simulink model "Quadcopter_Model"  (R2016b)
settings: Solver=VariableStepAuto  StartTime=0.0  StopTime=10.0  RelTol=1e-3
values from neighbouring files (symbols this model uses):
  g = 9.81    [modelParameters.m]
  If = 0.511    [modelParameters.m]
  Jreq = 4.2012e-05    [modelParameters.m]
  Jxx = 0.0218    [modelParameters.m]
  Jyy = 0.0277    [modelParameters.m]
  Jzz = 0.0332    [modelParameters.m]
  Kd = 1.8087e-07    [modelParameters.m]
  Kq = 96.3422    [modelParameters.m]
  Kt = 8.1558*10^-6    (= 8.1558e-06)    [modelParameters.m]
  Kv = 96.3422    [modelParameters.m]
  m = 1.19    [modelParameters.m]
  Pmax = 0.80    (= 0.8)    [modelParameters.m]
  Pmin = 0.40    (= 0.4)    [modelParameters.m]
  rhx = 0.016    [modelParameters.m]
  rhy = 0.016    [modelParameters.m]
  rhz = 0.003    [modelParameters.m]
  Rm = 0.2308    [modelParameters.m]
  Vb = 11.1    [modelParameters.m]

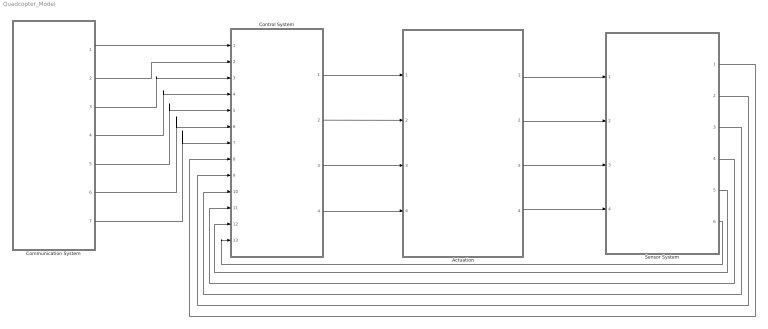
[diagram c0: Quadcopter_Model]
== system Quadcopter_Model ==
  Actuation : Subsystem
  Communication System : Subsystem
  Control System : Subsystem
  Sensor System : Subsystem
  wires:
  Control System/1(Rotor 0 Duty Cycle) -> Actuation/1(Rotor 0 Duty Cycle)
  Sensor System/6(Yaw rate (psi dot)) -> Control System/13(Yaw rate (psi dot))
  Sensor System/5(Roll rate (theta dot)) -> Control System/12(Roll rate (theta dot))
  Sensor System/4(Pitch rate (phi dot)) -> Control System/11(Pitch rate (phi dot))
  Sensor System/3(Yaw (psi)) -> Control System/10(Yaw (psi))
  Sensor System/2(Roll (theta)) -> Control System/9(Roll (theta))
  Sensor System/1(Pitch (phi)) -> Control System/8(Pitch (phi))
  Communication System/1(x_position) -> Control System/1(x position)
  Communication System/2(y_position) -> Control System/2(y position)
  Communication System/3(z_position) -> Control System/3(z position)
  Communication System/4(x_setpoint) -> Control System/4(x setpoint)
  Communication System/5(y_setpoint) -> Control System/5(y setpoint)
  Communication System/6(z_setpoint) -> Control System/6(z setpoint)
  Communication System/7(yaw_setpoint) -> Control System/7("Yaw setpoint ")
  Control System/2(Rotor 1 Duty Cycle) -> Actuation/2(Rotor 1 Duty Cycle)
  Control System/3(Rotor 2 Duty Cycle) -> Actuation/3(Rotor 2 Duty Cycle)
  Control System/4(Rotor 3 Duty Cycle) -> Actuation/4(Rotor 3 Duty Cycle)
  Actuation/1(B_omega) -> Sensor System/1(B_omega)
  Actuation/2(euler_angles) -> Sensor System/2(euler_angles)
  Actuation/3(B_vo) -> Sensor System/3(B_vo)
  Actuation/4(E_ro) -> Sensor System/4(E_ro)

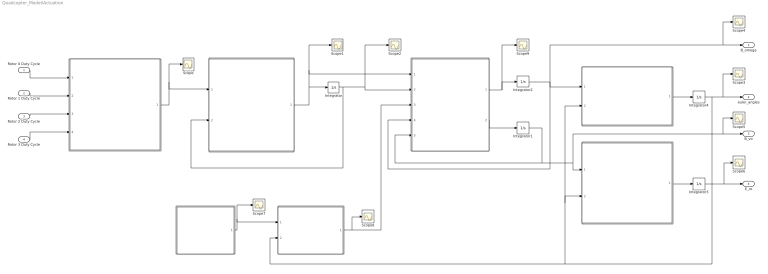
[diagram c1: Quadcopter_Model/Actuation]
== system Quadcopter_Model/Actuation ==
  Rotor 0 Duty Cycle : Inport
  Rotor 1 Duty Cycle : Inport  Port=2
  Rotor 2 Duty Cycle : Inport  Port=3
  Rotor 3 Duty Cycle : Inport  Port=4
  " " : MATLAB Function  TreatAsAtomicUnit=on
  " " : MATLAB Function  TreatAsAtomicUnit=on
  " " : MATLAB Function  TreatAsAtomicUnit=on
  " " : MATLAB Function  TreatAsAtomicUnit=on
  " " : MATLAB Function  TreatAsAtomicUnit=on
  " " : MATLAB Function  TreatAsAtomicUnit=on
  " " : MATLAB Function  TreatAsAtomicUnit=on
  Integrator{,1..3} (4 alike) : Integrator
  Integrator4 : Integrator  ContinuousStateAttributes=['phi' 'theta' 'psi']
  Scope{,1..9} (10 alike) : Scope
  B_omega : Outport
  euler_angles : Outport  Port=2
  B_vo : Outport  Port=3
  E_ro : Outport  Port=4
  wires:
  Rotor 3 Duty Cycle/1 -> " "/4(rotor_3_duty_cycle)
  Rotor 2 Duty Cycle/1 -> " "/3(rotor_2_duty_cycle)
  Rotor 1 Duty Cycle/1 -> " "/2(rotor_1_duty_cycle)
  Rotor 0 Duty Cycle/1 -> " "/1(rotor_0_duty_cycle)
  " "/1(Vb_eff) -> Scope/1, " "/1(Vb_eff)
  " "/1(angular_acceleration) -> Integrator/1, Scope1/1, " "/1(angular_acceleration)
  Integrator/1 -> Scope2/1, " "/2(angular_velocity), " "/2(angular_velocity)
  " "/1(B_omega_dot) -> Scope9/1, Integrator2/1
  " "/2(B_vo_dot) -> Integrator1/1
  Integrator2/1 -> Scope4/1, B_omega/1, " "/4(B_omega), " "/1(B_omega)
  Integrator1/1 -> " "/5(B_vo), " "/1(B_vo), B_vo/1, Scope5/1
  " "/1(euler_rates) -> Integrator4/1
  Integrator4/1 -> Scope3/1, euler_angles/1, " "/2(euler_angles), " "/2(euler_angles), " "/2(euler_angles)
  " "/1(E_Fg) -> Scope7/1, " "/1(E_Fg)
  " "/1(E_ro) -> Integrator3/1
  Integrator3/1 -> Scope6/1, E_ro/1
  " "/1(B_Fg) -> Scope8/1, " "/3(B_Fg)

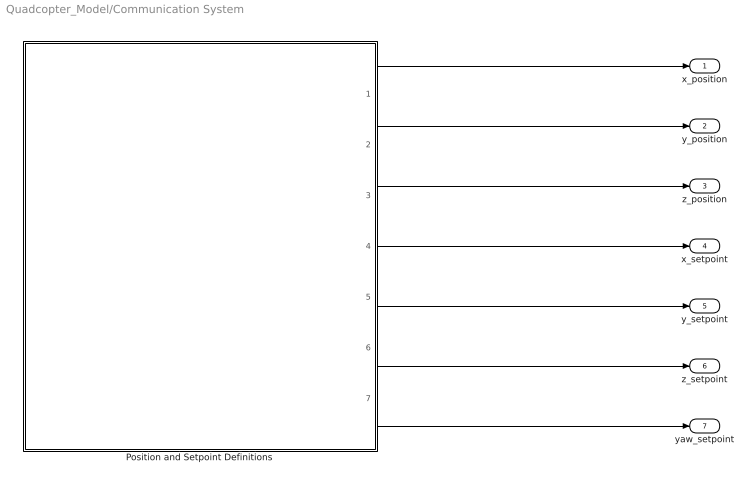
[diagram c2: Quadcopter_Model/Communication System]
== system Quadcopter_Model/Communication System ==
  Position and Setpoint Definitions : MATLAB Function  TreatAsAtomicUnit=on
  x_position : Outport
  y_position : Outport  Port=2
  z_position : Outport  Port=3
  x_setpoint : Outport  Port=4
  y_setpoint : Outport  Port=5
  z_setpoint : Outport  Port=6
  yaw_setpoint : Outport  Port=7
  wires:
  Position and Setpoint Definitions/7(yaw_setpoint) -> yaw_setpoint/1
  Position and Setpoint Definitions/6(z_setpoint) -> z_setpoint/1
  Position and Setpoint Definitions/5(y_setpoint) -> y_setpoint/1
  Position and Setpoint Definitions/4(x_setpoint) -> x_setpoint/1
  Position and Setpoint Definitions/3(z_position) -> z_position/1
  Position and Setpoint Definitions/2(y_position) -> y_position/1
  Position and Setpoint Definitions/1(x_position) -> x_position/1

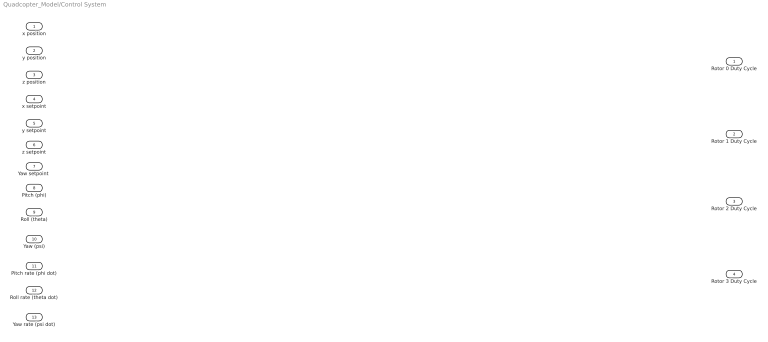
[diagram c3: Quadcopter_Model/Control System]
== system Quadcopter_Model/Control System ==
  x position : Inport
  y position : Inport  Port=2
  z position : Inport  Port=3
  x setpoint : Inport  Port=4
  y setpoint : Inport  Port=5
  z setpoint : Inport  Port=6
  "Yaw setpoint " : Inport  Port=7
  Pitch (phi) : Inport  Port=8
  Roll (theta) : Inport  Port=9
  Yaw (psi) : Inport  Port=10
  Pitch rate (phi dot) : Inport  Port=11
  Roll rate (theta dot) : Inport  Port=12
  Yaw rate (psi dot) : Inport  Port=13
  Rotor 0 Duty Cycle : Outport
  Rotor 1 Duty Cycle : Outport  Port=2
  Rotor 2 Duty Cycle : Outport  Port=3
  Rotor 3 Duty Cycle : Outport  Port=4

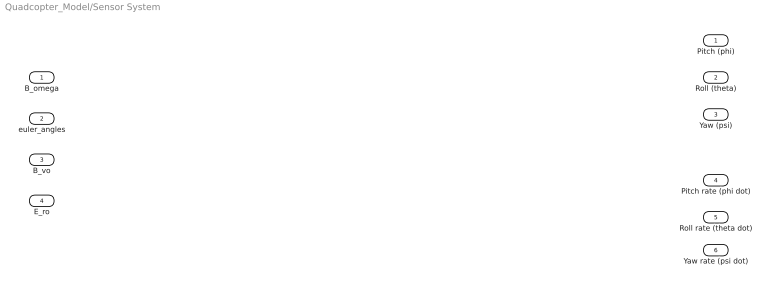
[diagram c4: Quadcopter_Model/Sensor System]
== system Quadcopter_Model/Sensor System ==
  B_omega : Inport
  euler_angles : Inport  Port=2
  B_vo : Inport  Port=3
  E_ro : Inport  Port=4
  Pitch (phi) : Outport
  Roll (theta) : Outport  Port=2
  Yaw (psi) : Outport  Port=3
  Pitch rate (phi dot) : Outport  Port=4
  Roll rate (theta dot) : Outport  Port=5
  Yaw rate (psi dot) : Outport  Port=6

== matlab function Quadcopter_Model/Actuation/



 ==
function E_Fg = gravity(  m, g)

E_Fg = [0; 0; m*g];

== matlab function Quadcopter_Model/Actuation/






 ==
function E_ro  = linear_body_earth_conversion(B_vo, euler_angles)

euler_rates = zeros(3,1);
E_ro = zeros(3,1);

phi = euler_angles(1);
theta = euler_angles(2);
psi = euler_angles(3);

Leb = [cos(theta)*cos(psi), sin(phi)*sin(theta)*cos(psi)-cos(phi)*sin(psi), cos(phi)*sin(theta)*cos(psi)+sin(phi)*sin(psi); ...
       cos(theta)*sin(psi), sin(phi)*sin(theta)*sin(psi)+cos(phi)*cos(psi), cos(phi)*sin(theta)*sin(psi)-sin(phi)*cos(psi); ...
           -sin(theta)    ,                sin(phi)*cos(theta)            ,                 cos(phi)*cos(theta)           ];

E_ro = Leb * B_vo;

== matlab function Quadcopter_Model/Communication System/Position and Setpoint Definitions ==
function [x_position, y_position, z_position, x_setpoint,...
    y_setpoint, z_setpoint, yaw_setpoint]= positionAndSetpointDefinitions

x_position = 0;
y_position = 0;
z_position = 0;
x_setpoint = 0;
y_setpoint = 0;
z_setpoint = 0;
yaw_setpoint = 0;

end

== matlab function Quadcopter_Model/Actuation/

 ==
function Vb_eff   = ESC(rotor_0_duty_cycle, rotor_1_duty_cycle, rotor_2_duty_cycle, rotor_3_duty_cycle, Pmin, Pmax, Vb)

% Define u_Pi for each of the rotors
u_P0 = (rotor_0_duty_cycle/100 - Pmin) / (Pmax - Pmin);
u_P1 = (rotor_1_duty_cycle/100 - Pmin) / (Pmax - Pmin);
u_P2 = (rotor_2_duty_cycle/100 - Pmin) / (Pmax - Pmin);
u_P3 = (rotor_3_duty_cycle/100 - Pmin) / (Pmax - Pmin);

% Determine the effective battery voltage from each ESC
Vb_eff_0 = u_P0 * Vb;
Vb_eff_1 = u_P1 * Vb;
Vb_eff_2 = u_P2 * Vb;
Vb_eff_3 = u_P3 * Vb;

Vb_eff = [Vb_eff_0, Vb_eff_1, Vb_eff_2, Vb_eff_3];

== matlab function Quadcopter_Model/Actuation/
 ==
function angular_acceleration  = motor(Vb_eff, angular_velocity, Rm, Kv, Kq, Kd, If, Jreq)

angular_acceleration = zeros(1,4);

% Define each motors effective battery voltage
Vb_eff_0 = Vb_eff(1);
Vb_eff_1 = Vb_eff(2);
Vb_eff_2 = Vb_eff(3);
Vb_eff_3 = Vb_eff(4);

% Determine the angular velocity of each rotor from feedback
w_0 = angular_velocity(1);
w_1 = angular_velocity(2);
w_2 = angular_velocity(3);
w_3 = angular_velocity(4);

% Determine angular acceleration of each rotor
w_0_dot = 1/(Jreq*Rm*Kq) * Vb_eff_0 - 1/(Jreq*Rm*Kq*Kv) * w_0 - 1/(Jreq*Kq)*If - (Kd/Jreq) * w_0^2;
w_1_dot = 1/(Jreq*Rm*Kq) * Vb_eff_1 - 1/(Jreq*Rm*Kq*Kv) * w_1 - 1/(Jreq*Kq)*If - (Kd/Jreq) * w_1^2;
w_2_dot = 1/(Jreq*Rm*Kq) * Vb_eff_2 - 1/(Jreq*Rm*Kq*Kv) * w_2 - 1/(Jreq*Kq)*If - (Kd/Jreq) * w_2^2;
w_3_dot = 1/(Jreq*Rm*Kq) * Vb_eff_3 - 1/(Jreq*Rm*Kq*Kv) * w_3 - 1/(Jreq*Kq)*If - (Kd/Jreq) * w_3^2;

angular_acceleration = [w_0_dot, w_1_dot, w_2_dot, w_3_dot];

== matlab function Quadcopter_Model/Actuation/







 ==
function [B_omega_dot, B_vo_dot]= rotor(angular_acceleration, angular_velocity, B_Fg, B_omega, B_vo, m, Kt, Kd, rhx, rhy, rhz, Jreq, Jxx, Jyy, Jzz)

B_vo_dot = zeros(3,1);
B_omega_dot = zeros(3,1);

% Create J vector
J = [Jxx,  0 ,  0 ; ...
      0 , Jyy,  0 ; ...
      0 ,  0 , Jzz;];

% Create r_hi vector
rh_0 = [-rhx; rhy; rhz];
rh_1 = [rhx; rhy; rhz];
rh_2 = [-rhx; -rhy; rhz];
rh_3 = [rhx; -rhy; rhz];

% Define vector from body frame origin to center of mass
br_oc = [0; 0; 0];

% Define 3x3 Identity Matrix
I = eye(3);

% Create gamma vectors
gamma_Ti = [0; 0; -1];
gamma_omega_03 = [0; 0; -1];  %Rotors 0 and 3 use this gamma_omega vector
gamma_omega_12 = [0; 0; 1]; %Rotors 1 and 2 use this gamma_omega vector

% Define angular velocities for each rotor
w_0 = angular_velocity(1);
w_1 = angular_velocity(2);
w_2 = angular_velocity(3);
w_3 = angular_velocity(4);

% Define angular acceleration for each rotor
w_0_dot = angular_acceleration(1);
w_1_dot = angular_acceleration(2);
w_2_dot = angular_acceleration(3);
w_3_dot = angular_acceleration(4);

% Define the rotor force in the z-direction from each rotor
B_Fr_0 = Kt * w_0 * w_0 * gamma_Ti;
B_Fr_1 = Kt * w_1 * w_1 * gamma_Ti;
B_Fr_2 = Kt * w_2 * w_2 * gamma_Ti;
B_Fr_3 = Kt * w_3 * w_3 * gamma_Ti;

% Sum up the rotor forces in the z-direction from each vector to get the
% total body force in the z-direction
B_Fr = B_Fr_0 + B_Fr_1 + B_Fr_2 + B_Fr_3;

% Define the in-plane drag and induced torque produced by each rotor
 B_Q_d0 = -1 * Kd * w_0 * w_0 * gamma_omega_03;
 B_Q_d1 = -1 * Kd * w_1 * w_1 * gamma_omega_12;
 B_Q_d2 = -1 * Kd * w_2 * w_2 * gamma_omega_12;
 B_Q_d3 = -1 * Kd * w_3 * w_3 * gamma_omega_03;

% Sum up the total in-plane drag and induced torque to get the total
% in-plane drag and induced torque on the body
B_Q_d = B_Q_d0 + B_Q_d1 + B_Q_d2 + B_Q_d3;

% Define the force lever arm torque created from the force produced by each
% rotor in the z-direction
B_Q_F0 = cross( rh_0, B_Fr_0 );
B_Q_F1 = cross( rh_1, B_Fr_1 );
B_Q_F2 = cross( rh_2, B_Fr_2 );
B_Q_F3 = cross( rh_3, B_Fr_3 );

B_Q_F = B_Q_F0 + B_Q_F1 + B_Q_F2 + B_Q_F3;

%Define the change in angular momentum torque produced by each rotor 
B_Q_L0 = -1 * Jreq * ( cross(B_omega, w_0 * gamma_omega_03) + w_0_dot * gamma_omega_03 );
B_Q_L1 = -1 * Jreq * ( cross(B_omega, w_1 * gamma_omega_12) + w_1_dot * gamma_omega_12 ); 
B_Q_L2 = -1 * Jreq * ( cross(B_omega, w_2 * gamma_omega_12) + w_2_dot * gamma_omega_12 ); 
B_Q_L3 = -1 * Jreq * ( cross(B_omega, w_3 * gamma_omega_03) + w_3_dot * gamma_omega_03 );

% Sum up the total change in angular momentum torque produced by each rotor
B_Q_L = B_Q_L0 + B_Q_L1 + B_Q_L2 + B_Q_L3;

% Define the total rotor system torque as the sum of the in-plane drag and
% induced torque, force lever arm torque, and change in angular momentum
% torques
B_Q = B_Q_d + B_Q_F + B_Q_L;

% Define the body forces in the z-direction from each vector to get the
% total body force in the z-direction
B_F = B_Fr + B_Fg; 

% Define the body frame linear velocities
B_vo_dot = (m*I)^(-1) * ( B_F - cross( B_omega, m*(B_vo + cross(B_omega, br_oc)) ) );

% Define the body frame angular velocities
B_omega_dot = J ^(-1) * ( B_Q - cross(B_omega, J * B_omega) - cross(br_oc, B_F) );

== matlab function Quadcopter_Model/Actuation/














 ==
function euler_rates = angular_body_earth_conversion(B_omega, euler_angles)

euler_rates = zeros(3,1);

phi = euler_angles(1);
theta = euler_angles(2);

Aeb = [1, sin(phi)*tan(theta), cos(phi)*tan(theta); ...
       0,     cos(phi)       ,        -sin(phi)   ; ...
       0,  sin(phi)/cos(theta), cos(phi)/cos(theta)];

   
euler_rates = Aeb * B_omega;

== matlab function Quadcopter_Model/Actuation/






















 ==
function B_Fg  = linear_earth_body_conversion(E_Fg, euler_angles)

euler_rates = zeros(3,1);
B_Fg = zeros(3,1);

phi = euler_angles(1);
theta = euler_angles(2);
psi = euler_angles(3);

Lbe = [             cos(theta)*cos(psi)              ,          cos(theta)*sin(psi)                  ,     -sin(theta)    ; ...
       sin(phi)*sin(theta)*cos(psi)-cos(phi)*sin(psi), sin(phi)*sin(theta)*sin(psi)+cos(phi)*cos(psi), sin(phi)*cos(theta); ...
       cos(phi)*sin(theta)*cos(psi)+sin(phi)*sin(psi), cos(phi)*sin(theta)*sin(psi)-sin(phi)*cos(psi), cos(phi)*cos(theta)];

B_Fg = Lbe * E_Fg;
